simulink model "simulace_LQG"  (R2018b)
settings: Solver=ode4  StartTime=0.0  StopTime=10.5  FixedStep=1e-3  RelTol=1e-3
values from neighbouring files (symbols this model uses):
  b_0 = (bn_0 + bp_0) / 2    [mainSkript_simulaceLQG.m]    (also in mainSkript_rovniceSystemu.m = (params.bp_0 + params.bn_0) / 2; mainSkript_overeniRovnic.m = 0; mainSkript_LQGexperiment.m; mainSkript_LQGexperiment_integral.m)
  b_1 = params.b_1    [mainSkript_simulaceLQG.m]    (also in mainSkript_rovniceSystemu.m; mainSkript_overeniRovnic.m; mainSkript_kyvadlaNajednouOdhad.m; mainSkript_LQGexperiment.m)
  b_2 = params.b_2    [mainSkript_simulaceLQG.m]    (also in mainSkript_rovniceSystemu.m; mainSkript_overeniRovnic.m; mainSkript_kyvadlaNajednouOdhad.m; mainSkript_LQGexperiment.m)
  g = 9.81    [mainSkript_simulaceLQG.m]    (also in mainSkript_rovniceSystemu.m; mainSkript_overeniRovnic.m; mainSkript_estimaceVozik.m; mainSkript_odhadKyvadlaZvlast.m)
  I_1 = params.I_1    [mainSkript_simulaceLQG.m]    (also in mainSkript_rovniceSystemu.m; mainSkript_overeniRovnic.m; mainSkript_kyvadlaNajednouOdhad.m; mainSkript_LQGexperiment.m)
  I_2 = params.I_2    [mainSkript_simulaceLQG.m]    (also in mainSkript_rovniceSystemu.m; mainSkript_overeniRovnic.m; mainSkript_kyvadlaNajednouOdhad.m; mainSkript_LQGexperiment.m)
  K = lqr(sysd, Qk, Rk)    [mainSkript_simulaceLQG.m]    (also in makeFBL.m = [0; -d_2*g*sin(th_1); -d_3*g*sin(th_2)]; mainSkript_LQGexperiment.m = lqr(sysd, Q, R); mainSkript_LQGexperiment_integral.m = lqr(sysd, Q, R); mainSkript_pocitaniTVLQR_simplified.m = zeros(N + 1, n_sts))
  l_1 = params.l_1    [mainSkript_simulaceLQG.m]    (also in mainSkript_rovniceSystemu.m; mainSkript_overeniRovnic.m; odhadovane_parametry.m = 0.134; mainSkript_kyvadlaNajednouOdhad.m)
  L_1 = params.L_1    [mainSkript_simulaceLQG.m]    (also in mainSkript_rovniceSystemu.m; mainSkript_overeniRovnic.m; odhadovane_parametry.m = 0.228; mainSkript_kyvadlaNajednouOdhad.m)
  l_2 = params.l_2    [mainSkript_simulaceLQG.m]    (also in mainSkript_rovniceSystemu.m; mainSkript_overeniRovnic.m; odhadovane_parametry.m = 0.112; mainSkript_kyvadlaNajednouOdhad.m)
  m_0 = params.m_0    [mainSkript_simulaceLQG.m]    (also in mainSkript_rovniceSystemu.m; mainSkript_overeniRovnic.m; mainSkript_LQGexperiment.m; mainSkript_LQGexperiment_integral.m)
  m_1 = params.m_1    [mainSkript_simulaceLQG.m]    (also in mainSkript_rovniceSystemu.m; mainSkript_overeniRovnic.m; mainSkript_kyvadlaNajednouOdhad.m; mainSkript_LQGexperiment.m)
  m_2 = params.m_2    [mainSkript_simulaceLQG.m]    (also in mainSkript_rovniceSystemu.m; mainSkript_overeniRovnic.m; mainSkript_kyvadlaNajednouOdhad.m; mainSkript_LQGexperiment.m)
  N = N * Cref'    [mainSkript_simulaceLQG.m]    (also in mainSkript_tvorbaTrajektorii.m = 100; mainSkript_pocitaniTVLQR_simplified.m = floor( length(time) / krok ))
  q_0 = [0 th1_0 th2_0 0 dth1_0 dth2_0]    [mainSkript_simulaceLQG.m]    (also in mainSkript_kyvadlaNajednouOdhad.m = cell(1, k); mainSkript_LQGexperiment.m = zeros(6,1); mainSkript_LQGexperiment_integral.m = zeros(6,1); mainSkript_modifikaceParametru.m = [0 pi pi 0 0 0])
  Ts = 1e-3    (= 0.001)    [mainSkript_simulaceLQG.m]    (also in mainSkript_rovniceSystemu.m; mainSkript_LQGexperiment.m; mainSkript_LQGexperiment_integral.m; mainSkript_modifikaceParametru.m)
undefined symbols (not defined in the file or in its folder): DiscIntNeverNeededParam
libraries: sharedTrackingLibrary x1, simulink x1

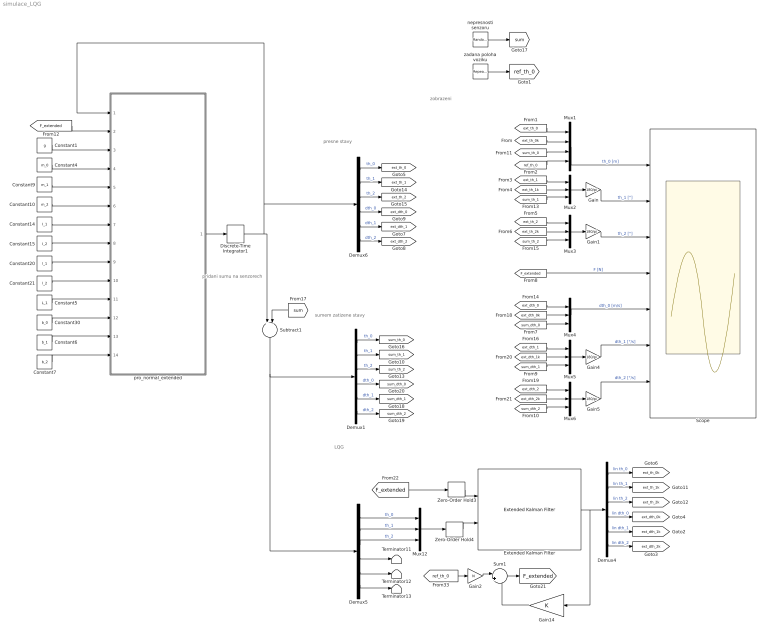
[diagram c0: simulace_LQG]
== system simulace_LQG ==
  note: sumem zatizene stavy
  note: presne stavy
  note: zobrazeni
  note: pridani sumu na senzorech
  note: LQG
  Constant1 : Constant  Value=g
  Constant10 : Constant  Value=m_2
  Constant14 : Constant  Value=I_1
  Constant15 : Constant  Value=I_2
  Constant20 : Constant  Value=l_1
  Constant21 : Constant  Value=l_2
  Constant30 : Constant  Value=b_0
  Constant4 : Constant  Value=m_0
  Constant5 : Constant  Value=L_1
  Constant6 : Constant  Value=b_1
  Constant7 : Constant  Value=b_2
  Constant9 : Constant  Value=m_1
  Demux{1,4..6} (4 alike) : Demux  Outputs=6
  Discrete-Time Integrator1 : DiscreteIntegrator  InitialCondition=q_0  SampleTime=Ts  ICPrevOutput=DiscIntNeverNeededParam  ICPrevScaledInput=DiscIntNeverNeededParam
  Extended Kalman Filter : sharedTrackingLibrary/Extended Kalman Filter  StateTransitionFcn=nonLinKalmFcn  HasStateTransitionJacobianFcn=on  StateTransitionJacobianFcn=countJacobDIP  HasAdditiveProcessNoise=Additive  ProcessNoise=Q_kalm  HasTimeVaryingProcessNoise=off  HasStateTransitionFcnExtraArgument=1  InitialState=q_0  InitialStateCovariance=1e-3*eye(6)  MeasurementFcn1=mereniStavuKalm  HasMeasurementJacobianFcn1=off  HasMeasurementEnablePort1=off  HasAdditiveMeasurementNoise1=Additive  MeasurementNoise1=R_kalm  HasTimeVaryingMeasurementNoise1=off  HasMeasurementFcnExtraArgument1=0  MeasurementFcn2=myMeasurementFcn  HasMeasurementJacobianFcn2=off  HasMeasurementEnablePort2=off  HasAdditiveMeasurementNoise2=Additive  MeasurementNoise2=1  HasTimeVaryingMeasurementNoise2=off  HasMeasurementFcnExtraArgument2=0  MeasurementFcn3=myMeasurementFcn  HasMeasurementJacobianFcn3=off  HasMeasurementEnablePort3=off  HasAdditiveMeasurementNoise3=Additive  MeasurementNoise3=1  HasTimeVaryingMeasurementNoise3=off  HasMeasurementFcnExtraArgument3=0  MeasurementFcn4=myMeasurementFcn  HasMeasurementJacobianFcn4=off  HasMeasurementEnablePort4=off  HasAdditiveMeasurementNoise4=Additive  MeasurementNoise4=1  HasTimeVaryingMeasurementNoise4=off  HasMeasurementFcnExtraArgument4=0  MeasurementFcn5=myMeasurementFcn  HasMeasurementJacobianFcn5=off  HasMeasurementEnablePort5=off  HasAdditiveMeasurementNoise5=Additive  MeasurementNoise5=1  HasTimeVaryingMeasurementNoise5=off  HasMeasurementFcnExtraArgument5=0  EnableMultirate=off  StateTransitionFcnSampleTime=1  MeasurementFcn1SampleTime=1  MeasurementFcn2SampleTime=1  MeasurementFcn3SampleTime=1  MeasurementFcn4SampleTime=1  MeasurementFcn5SampleTime=1  UseCurrentEstimator=on  OutputStateCovariance=off  DataType=double  SampleTime=1e-3  NumberOfMeasurements=1
  Gain{,1,4..5} (4 alike) : Gain  Gain=180/pi
  Gain14 : Gain  Gain=K  Multiplication=Matrix(K*u) (u vector)
  Gain2 : Gain  Gain=N
  Mux1 : Mux
  Mux{2..6,12} (6 alike) : Mux  Inputs=3
  Scope : Scope  NumInputPorts=7
  Subtract1 : Sum  Inputs=+-
  Sum1 : Sum  Inputs=|+-
  Terminator11 : Terminator
  Terminator12 : Terminator
  Terminator13 : Terminator
  Zero-Order Hold3 : ZeroOrderHold  SampleTime=1e-3
  Zero-Order Hold4 : ZeroOrderHold  SampleTime=1e-3
  nepresnosti senzoru : RandomNumber  Mean=zeros(6,1)  Variance=[1e-5 .* ones(6,1)]  SampleTime=1e-3
  pro_normal_extended : MATLAB Function  TreatAsAtomicUnit=on
  zadana poloha voziku : simulink/Sources/Repeating Sequence Stair  OutValues=[0 0.1 -0.1]  tsamp=5  OutMin=[]  OutMax=[]  OutDataTypeStr=double  OutputDataTypeScalingMode=double  OutDataType=fixdt(0,8)  ConRadixGroup=Best Precision: Vector-wise  OutScaling=2^-12
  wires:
  [F_extended] -> Zero-Order Hold3/1
  Demux4/1 -> [ext_th_0k]  "lin th_0"
  Demux4/4 -> [ext_dth_0k]  "lin dth_0"
  Demux4/5 -> [ext_dth_1k]  "lin dth_1"
  Demux4/3 -> [ext_th_2k]  "lin th_2"
  Demux4/2 -> [ext_th_1k]  "lin th_1"
  Demux4/6 -> [ext_dth_2k]  "lin dth_2"
  Extended Kalman Filter/1 -> Gain14/1, Demux4/1
  Constant30/1 -> pro_normal_extended/12(b_0)
  Constant7/1 -> pro_normal_extended/14(b_2)
  Constant5/1 -> pro_normal_extended/11(L_1)
  Demux6/2 -> [ext_th_1]  "th_1"
  Constant1/1 -> pro_normal_extended/3(g)
  Constant21/1 -> pro_normal_extended/10(l_2)
  Demux6/3 -> [ext_th_2]  "th_2"
  Constant6/1 -> pro_normal_extended/13(b_1)
  Demux6/1 -> [ext_th_0]  "th_0"
  pro_normal_extended/1(dx) -> Discrete-Time Integrator1/1
  Constant14/1 -> pro_normal_extended/7(I_1)
  Constant15/1 -> pro_normal_extended/8(I_2)
  Constant4/1 -> pro_normal_extended/4(m_0)
  Constant9/1 -> pro_normal_extended/5(m_1)
  Constant20/1 -> pro_normal_extended/9(l_1)
  Discrete-Time Integrator1/1 -> Demux6/1, pro_normal_extended/1(y), Subtract1/1
  Constant10/1 -> pro_normal_extended/6(m_2)
  [F_extended] -> pro_normal_extended/2(u)
  nepresnosti senzoru/1 -> [sum]
  [sum] -> Subtract1/2
  zadana poloha voziku/1 -> [ref_th_0]
  [ext_th_1] -> Mux2/1
  [ext_th_1k] -> Mux2/2
  [ext_th_2k] -> Mux3/2
  [ext_th_2] -> Mux3/1
  Mux1/1 -> Scope/1  "th_0 [m]"
  Mux2/1 -> Gain/1
  Mux3/1 -> Gain1/1
  [F_extended] -> Scope/4  "F [N]"
  Gain/1 -> Scope/2  "th_1 [°]"
  Gain1/1 -> Scope/3  "th_2 [°]"
  [ext_th_0] -> Mux1/1
  [ext_th_0k] -> Mux1/2
  [ref_th_0] -> Gain2/1
  Gain2/1 -> Sum1/1
  Gain14/1 -> Sum1/2
  Zero-Order Hold3/1 -> Extended Kalman Filter/1
  Zero-Order Hold4/1 -> Extended Kalman Filter/2
  Mux6/1 -> Gain5/1
  Gain4/1 -> Scope/6  "dth_1 [°/s]"
  Gain5/1 -> Scope/7  "dth_2 [°/s]"
  Demux6/4 -> [ext_dth_0]  "dth_0"
  Demux6/5 -> [ext_dth_1]  "dth_1"
  Demux6/6 -> [ext_dth_2]  "dth_2"
  Mux4/1 -> Scope/5  "dth_0 [m/s]"
  Demux1/6 -> [sum_dth_2]  "dth_2"
  Demux1/5 -> [sum_dth_1]  "dth_1"
  Demux1/4 -> [sum_dth_0]  "dth_0"
  Demux1/1 -> [sum_th_0]  "th_0"
  Demux1/3 -> [sum_th_2]  "th_2"
  Demux1/2 -> [sum_th_1]  "th_1"
  [ref_th_0] -> Mux1/4
  [sum_th_0] -> Mux1/3
  [sum_th_1] -> Mux2/3
  [sum_th_2] -> Mux3/3
  [ext_dth_0] -> Mux4/1
  [sum_dth_0] -> Mux4/3
  [ext_dth_0k] -> Mux4/2
  [ext_dth_1] -> Mux5/1
  [sum_dth_1] -> Mux5/3
  [ext_dth_1k] -> Mux5/2
  Mux5/1 -> Gain4/1
  [ext_dth_2] -> Mux6/1
  [sum_dth_2] -> Mux6/3
  [ext_dth_2k] -> Mux6/2
  Sum1/1 -> [F_extended]
  Demux5/2 -> Mux12/2  "th_1"
  Demux5/3 -> Mux12/3  "th_2"
  Demux5/6 -> Terminator13/1
  Demux5/1 -> Mux12/1  "th_0"
  Demux5/4 -> Terminator11/1
  Demux5/5 -> Terminator12/1
  Mux12/1 -> Zero-Order Hold4/1
  Subtract1/1 -> Demux5/1, Demux1/1

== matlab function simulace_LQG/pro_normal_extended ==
function dx = PohybovaRceDIP_basic(y, u, g, m_0, m_1, m_2, I_1, I_2, l_1, l_2, L_1, b_0, b_1, b_2)
%PohybovaRceDIP_basic: Pohybova rovnice dvojiteho kyvadla

dx = zeros(6, 1); % definovani sloupcoveho vektoru derivaci stavu 

dx(1) = conj(y(4)); 
dx(2) = conj(y(5)); 
dx(3) = conj(y(6)); 
dx(4) = conj(y(6))*((b_2*(L_1^2*l_2*m_2^2*cos(y(3)) + I_1*l_2*m_2*cos(y(3)) - L_1^2*l_2*m_2^2*cos(y(2) - y(3))*cos(y(2)) + l_1^2*l_2*m_1*m_2*cos(y(3)) - L_1*l_1*l_2*m_1*m_2*cos(y(2) - y(3))*cos(y(2))))/(I_2*L_1^2*m_2^2 + I_2*l_1^2*m_1^2 + I_1*l_2^2*m_2^2 + I_1*I_2*m_0 + I_1*I_2*m_1 + I_1*I_2*m_2 + L_1^2*l_2^2*m_2^3 + L_1^2*l_2^2*m_0*m_2^2 + L_1^2*l_2^2*m_1*m_2^2 - L_1^2*l_2^2*m_2^3*cos(y(2) - y(3))^2 + I_2*L_1^2*m_0*m_2 + I_2*L_1^2*m_1*m_2 + l_1^2*l_2^2*m_1*m_2^2 + l_1^2*l_2^2*m_1^2*m_2 + I_2*l_1^2*m_0*m_1 + I_1*l_2^2*m_0*m_2 + I_1*l_2^2*m_1*m_2 + I_2*l_1^2*m_1*m_2 - I_2*L_1^2*m_2^2*cos(y(2))^2 - I_2*l_1^2*m_1^2*cos(y(2))^2 - I_1*l_2^2*m_2^2*cos(y(3))^2 - L_1^2*l_2^2*m_2^3*cos(y(2))^2 - L_1^2*l_2^2*m_2^3*cos(y(3))^2 + l_1^2*l_2^2*m_0*m_1*m_2 - l_1^2*l_2^2*m_1^2*m_2*cos(y(2))^2 - l_1^2*l_2^2*m_1*m_2^2*cos(y(3))^2 - L_1^2*l_2^2*m_0*m_2^2*cos(y(2) - y(3))^2 - L_1^2*l_2^2*m_1*m_2^2*cos(y(2) - y(3))^2 - 2*L_1*l_1*l_2^2*m_1*m_2^2*cos(y(2))^2 + 2*L_1^2*l_2^2*m_2^3*cos(y(2) - y(3))*cos(y(2))*cos(y(3)) - 2*I_2*L_1*l_1*m_1*m_2*cos(y(2))^2 + 2*L_1*l_1*l_2^2*m_1*m_2^2*cos(y(2) - y(3))*cos(y(2))*cos(y(3))) - ((b_2 - L_1*l_2*m_2*sin(y(2) - y(3))*y(6))*(L_1*l_2^2*m_2^2*cos(y(2)) + I_2*L_1*m_2*cos(y(2)) + I_2*l_1*m_1*cos(y(2)) - L_1*l_2^2*m_2^2*cos(y(2) - y(3))*cos(y(3)) + l_1*l_2^2*m_1*m_2*cos(y(2))))/(I_2*L_1^2*m_2^2 + I_2*l_1^2*m_1^2 + I_1*l_2^2*m_2^2 + I_1*I_2*m_0 + I_1*I_2*m_1 + I_1*I_2*m_2 + L_1^2*l_2^2*m_2^3 + L_1^2*l_2^2*m_0*m_2^2 + L_1^2*l_2^2*m_1*m_2^2 - L_1^2*l_2^2*m_2^3*cos(y(2) - y(3))^2 + I_2*L_1^2*m_0*m_2 + I_2*L_1^2*m_1*m_2 + l_1^2*l_2^2*m_1*m_2^2 + l_1^2*l_2^2*m_1^2*m_2 + I_2*l_1^2*m_0*m_1 + I_1*l_2^2*m_0*m_2 + I_1*l_2^2*m_1*m_2 + I_2*l_1^2*m_1*m_2 - I_2*L_1^2*m_2^2*cos(y(2))^2 - I_2*l_1^2*m_1^2*cos(y(2))^2 - I_1*l_2^2*m_2^2*cos(y(3))^2 - L_1^2*l_2^2*m_2^3*cos(y(2))^2 - L_1^2*l_2^2*m_2^3*cos(y(3))^2 + l_1^2*l_2^2*m_0*m_1*m_2 - l_1^2*l_2^2*m_1^2*m_2*cos(y(2))^2 - l_1^2*l_2^2*m_1*m_2^2*cos(y(3))^2 - L_1^2*l_2^2*m_0*m_2^2*cos(y(2) - y(3))^2 - L_1^2*l_2^2*m_1*m_2^2*cos(y(2) - y(3))^2 - 2*L_1*l_1*l_2^2*m_1*m_2^2*cos(y(2))^2 + 2*L_1^2*l_2^2*m_2^3*cos(y(2) - y(3))*cos(y(2))*cos(y(3)) - 2*I_2*L_1*l_1*m_1*m_2*cos(y(2))^2 + 2*L_1*l_1*l_2^2*m_1*m_2^2*cos(y(2) - y(3))*cos(y(2))*cos(y(3))) + (l_2*m_2*y(6)*sin(y(3))*(I_1*I_2 + L_1^2*l_2^2*m_2^2 + I_2*L_1^2*m_2 + I_2*l_1^2*m_1 + I_1*l_2^2*m_2 - L_1^2*l_2^2*m_2^2*cos(y(2) - y(3))^2 + l_1^2*l_2^2*m_1*m_2))/(I_2*L_1^2*m_2^2 + I_2*l_1^2*m_1^2 + I_1*l_2^2*m_2^2 + I_1*I_2*m_0 + I_1*I_2*m_1 + I_1*I_2*m_2 + L_1^2*l_2^2*m_2^3 + L_1^2*l_2^2*m_0*m_2^2 + L_1^2*l_2^2*m_1*m_2^2 - L_1^2*l_2^2*m_2^3*cos(y(2) - y(3))^2 + I_2*L_1^2*m_0*m_2 + I_2*L_1^2*m_1*m_2 + l_1^2*l_2^2*m_1*m_2^2 + l_1^2*l_2^2*m_1^2*m_2 + I_2*l_1^2*m_0*m_1 + I_1*l_2^2*m_0*m_2 + I_1*l_2^2*m_1*m_2 + I_2*l_1^2*m_1*m_2 - I_2*L_1^2*m_2^2*cos(y(2))^2 - I_2*l_1^2*m_1^2*cos(y(2))^2 - I_1*l_2^2*m_2^2*cos(y(3))^2 - L_1^2*l_2^2*m_2^3*cos(y(2))^2 - L_1^2*l_2^2*m_2^3*cos(y(3))^2 + l_1^2*l_2^2*m_0*m_1*m_2 - l_1^2*l_2^2*m_1^2*m_2*cos(y(2))^2 - l_1^2*l_2^2*m_1*m_2^2*cos(y(3))^2 - L_1^2*l_2^2*m_0*m_2^2*cos(y(2) - y(3))^2 - L_1^2*l_2^2*m_1*m_2^2*cos(y(2) - y(3))^2 - 2*L_1*l_1*l_2^2*m_1*m_2^2*cos(y(2))^2 + 2*L_1^2*l_2^2*m_2^3*cos(y(2) - y(3))*cos(y(2))*cos(y(3)) - 2*I_2*L_1*l_1*m_1*m_2*cos(y(2))^2 + 2*L_1*l_1*l_2^2*m_1*m_2^2*cos(y(2) - y(3))*cos(y(2))*cos(y(3)))) + conj(y(5))*(((b_1 + b_2)*(L_1*l_2^2*m_2^2*cos(y(2)) + I_2*L_1*m_2*cos(y(2)) + I_2*l_1*m_1*cos(y(2)) - L_1*l_2^2*m_2^2*cos(y(2) - y(3))*cos(y(3)) + l_1*l_2^2*m_1*m_2*cos(y(2))))/(I_2*L_1^2*m_2^2 + I_2*l_1^2*m_1^2 + I_1*l_2^2*m_2^2 + I_1*I_2*m_0 + I_1*I_2*m_1 + I_1*I_2*m_2 + L_1^2*l_2^2*m_2^3 + L_1^2*l_2^2*m_0*m_2^2 + L_1^2*l_2^2*m_1*m_2^2 - L_1^2*l_2^2*m_2^3*cos(y(2) - y(3))^2 + I_2*L_1^2*m_0*m_2 + I_2*L_1^2*m_1*m_2 + l_1^2*l_2^2*m_1*m_2^2 + l_1^2*l_2^2*m_1^2*m_2 + I_2*l_1^2*m_0*m_1 + I_1*l_2^2*m_0*m_2 + I_1*l_2^2*m_1*m_2 + I_2*l_1^2*m_1*m_2 - I_2*L_1^2*m_2^2*cos(y(2))^2 - I_2*l_1^2*m_1^2*cos(y(2))^2 - I_1*l_2^2*m_2^2*cos(y(3))^2 - L_1^2*l_2^2*m_2^3*cos(y(2))^2 - L_1^2*l_2^2*m_2^3*cos(y(3))^2 + l_1^2*l_2^2*m_0*m_1*m_2 - l_1^2*l_2^2*m_1^2*m_2*cos(y(2))^2 - l_1^2*l_2^2*m_1*m_2^2*cos(y(3))^2 - L_1^2*l_2^2*m_0*m_2^2*cos(y(2) - y(3))^2 - L_1^2*l_2^2*m_1*m_2^2*cos(y(2) - y(3))^2 - 2*L_1*l_1*l_2^2*m_1*m_2^2*cos(y(2))^2 + 2*L_1^2*l_2^2*m_2^3*cos(y(2) - y(3))*cos(y(2))*cos(y(3)) - 2*I_2*L_1*l_1*m_1*m_2*cos(y(2))^2 + 2*L_1*l_1*l_2^2*m_1*m_2^2*cos(y(2) - y(3))*cos(y(2))*cos(y(3))) - ((b_2 + L_1*l_2*m_2*sin(y(2) - y(3))*y(5))*(L_1^2*l_2*m_2^2*cos(y(3)) + I_1*l_2*m_2*cos(y(3)) - L_1^2*l_2*m_2^2*cos(y(2) - y(3))*cos(y(2)) + l_1^2*l_2*m_1*m_2*cos(y(3)) - L_1*l_1*l_2*m_1*m_2*cos(y(2) - y(3))*cos(y(2))))/(I_2*L_1^2*m_2^2 + I_2*l_1^2*m_1^2 + I_1*l_2^2*m_2^2 + I_1*I_2*m_0 + I_1*I_2*m_1 + I_1*I_2*m_2 + L_1^2*l_2^2*m_2^3 + L_1^2*l_2^2*m_0*m_2^2 + L_1^2*l_2^2*m_1*m_2^2 - L_1^2*l_2^2*m_2^3*cos(y(2) - y(3))^2 + I_2*L_1^2*m_0*m_2 + I_2*L_1^2*m_1*m_2 + l_1^2*l_2^2*m_1*m_2^2 + l_1^2*l_2^2*m_1^2*m_2 + I_2*l_1^2*m_0*m_1 + I_1*l_2^2*m_0*m_2 + I_1*l_2^2*m_1*m_2 + I_2*l_1^2*m_1*m_2 - I_2*L_1^2*m_2^2*cos(y(2))^2 - I_2*l_1^2*m_1^2*cos(y(2))^2 - I_1*l_2^2*m_2^2*cos(y(3))^2 - L_1^2*l_2^2*m_2^3*cos(y(2))^2 - L_1^2*l_2^2*m_2^3*cos(y(3))^2 + l_1^2*l_2^2*m_0*m_1*m_2 - l_1^2*l_2^2*m_1^2*m_2*cos(y(2))^2 - l_1^2*l_2^2*m_1*m_2^2*cos(y(3))^2 - L_1^2*l_2^2*m_0*m_2^2*cos(y(2) - y(3))^2 - L_1^2*l_2^2*m_1*m_2^2*cos(y(2) - y(3))^2 - 2*L_1*l_1*l_2^2*m_1*m_2^2*cos(y(2))^2 + 2*L_1^2*l_2^2*m_2^3*cos(y(2) - y(3))*cos(y(2))*cos(y(3)) - 2*I_2*L_1*l_1*m_1*m_2*cos(y(2))^2 + 2*L_1*l_1*l_2^2*m_1*m_2^2*cos(y(2) - y(3))*cos(y(2))*cos(y(3))) + (y(5)*sin(y(2))*(L_1*m_2 + l_1*m_1)*(I_1*I_2 + L_1^2*l_2^2*m_2^2 + I_2*L_1^2*m_2 + I_2*l_1^2*m_1 + I_1*l_2^2*m_2 - L_1^2*l_2^2*m_2^2*cos(y(2) - y(3))^2 + l_1^2*l_2^2*m_1*m_2))/(I_2*L_1^2*m_2^2 + I_2*l_1^2*m_1^2 + I_1*l_2^2*m_2^2 + I_1*I_2*m_0 + I_1*I_2*m_1 + I_1*I_2*m_2 + L_1^2*l_2^2*m_2^3 + L_1^2*l_2^2*m_0*m_2^2 + L_1^2*l_2^2*m_1*m_2^2 - L_1^2*l_2^2*m_2^3*cos(y(2) - y(3))^2 + I_2*L_1^2*m_0*m_2 + I_2*L_1^2*m_1*m_2 + l_1^2*l_2^2*m_1*m_2^2 + l_1^2*l_2^2*m_1^2*m_2 + I_2*l_1^2*m_0*m_1 + I_1*l_2^2*m_0*m_2 + I_1*l_2^2*m_1*m_2 + I_2*l_1^2*m_1*m_2 - I_2*L_1^2*m_2^2*cos(y(2))^2 - I_2*l_1^2*m_1^2*cos(y(2))^2 - I_1*l_2^2*m_2^2*cos(y(3))^2 - L_1^2*l_2^2*m_2^3*cos(y(2))^2 - L_1^2*l_2^2*m_2^3*cos(y(3))^2 + l_1^2*l_2^2*m_0*m_1*m_2 - l_1^2*l_2^2*m_1^2*m_2*cos(y(2))^2 - l_1^2*l_2^2*m_1*m_2^2*cos(y(3))^2 - L_1^2*l_2^2*m_0*m_2^2*cos(y(2) - y(3))^2 - L_1^2*l_2^2*m_1*m_2^2*cos(y(2) - y(3))^2 - 2*L_1*l_1*l_2^2*m_1*m_2^2*cos(y(2))^2 + 2*L_1^2*l_2^2*m_2^3*cos(y(2) - y(3))*cos(y(2))*cos(y(3)) - 2*I_2*L_1*l_1*m_1*m_2*cos(y(2))^2 + 2*L_1*l_1*l_2^2*m_1*m_2^2*cos(y(2) - y(3))*cos(y(2))*cos(y(3)))) + (u*(I_1*I_2 + L_1^2*l_2^2*m_2^2 + I_2*L_1^2*m_2 + I_2*l_1^2*m_1 + I_1*l_2^2*m_2 - L_1^2*l_2^2*m_2^2*cos(y(2) - y(3))^2 + l_1^2*l_2^2*m_1*m_2))/(I_2*L_1^2*m_2^2 + I_2*l_1^2*m_1^2 + I_1*l_2^2*m_2^2 + I_1*I_2*m_0 + I_1*I_2*m_1 + I_1*I_2*m_2 + L_1^2*l_2^2*m_2^3 + L_1^2*l_2^2*m_0*m_2^2 + L_1^2*l_2^2*m_1*m_2^2 - L_1^2*l_2^2*m_2^3*cos(y(2) - y(3))^2 + I_2*L_1^2*m_0*m_2 + I_2*L_1^2*m_1*m_2 + l_1^2*l_2^2*m_1*m_2^2 + l_1^2*l_2^2*m_1^2*m_2 + I_2*l_1^2*m_0*m_1 + I_1*l_2^2*m_0*m_2 + I_1*l_2^2*m_1*m_2 + I_2*l_1^2*m_1*m_2 - I_2*L_1^2*m_2^2*cos(y(2))^2 - I_2*l_1^2*m_1^2*cos(y(2))^2 - I_1*l_2^2*m_2^2*cos(y(3))^2 - L_1^2*l_2^2*m_2^3*cos(y(2))^2 - L_1^2*l_2^2*m_2^3*cos(y(3))^2 + l_1^2*l_2^2*m_0*m_1*m_2 - l_1^2*l_2^2*m_1^2*m_2*cos(y(2))^2 - l_1^2*l_2^2*m_1*m_2^2*cos(y(3))^2 - L_1^2*l_2^2*m_0*m_2^2*cos(y(2) - y(3))^2 - L_1^2*l_2^2*m_1*m_2^2*cos(y(2) - y(3))^2 - 2*L_1*l_1*l_2^2*m_1*m_2^2*cos(y(2))^2 + 2*L_1^2*l_2^2*m_2^3*cos(y(2) - y(3))*cos(y(2))*cos(y(3)) - 2*I_2*L_1*l_1*m_1*m_2*cos(y(2))^2 + 2*L_1*l_1*l_2^2*m_1*m_2^2*cos(y(2) - y(3))*cos(y(2))*cos(y(3))) - (b_0*conj(y(4))*(I_1*I_2 + L_1^2*l_2^2*m_2^2 + I_2*L_1^2*m_2 + I_2*l_1^2*m_1 + I_1*l_2^2*m_2 - L_1^2*l_2^2*m_2^2*cos(y(2) - y(3))^2 + l_1^2*l_2^2*m_1*m_2))/(I_2*L_1^2*m_2^2 + I_2*l_1^2*m_1^2 + I_1*l_2^2*m_2^2 + I_1*I_2*m_0 + I_1*I_2*m_1 + I_1*I_2*m_2 + L_1^2*l_2^2*m_2^3 + L_1^2*l_2^2*m_0*m_2^2 + L_1^2*l_2^2*m_1*m_2^2 - L_1^2*l_2^2*m_2^3*cos(y(2) - y(3))^2 + I_2*L_1^2*m_0*m_2 + I_2*L_1^2*m_1*m_2 + l_1^2*l_2^2*m_1*m_2^2 + l_1^2*l_2^2*m_1^2*m_2 + I_2*l_1^2*m_0*m_1 + I_1*l_2^2*m_0*m_2 + I_1*l_2^2*m_1*m_2 + I_2*l_1^2*m_1*m_2 - I_2*L_1^2*m_2^2*cos(y(2))^2 - I_2*l_1^2*m_1^2*cos(y(2))^2 - I_1*l_2^2*m_2^2*cos(y(3))^2 - L_1^2*l_2^2*m_2^3*cos(y(2))^2 - L_1^2*l_2^2*m_2^3*cos(y(3))^2 + l_1^2*l_2^2*m_0*m_1*m_2 - l_1^2*l_2^2*m_1^2*m_2*cos(y(2))^2 - l_1^2*l_2^2*m_1*m_2^2*cos(y(3))^2 - L_1^2*l_2^2*m_0*m_2^2*cos(y(2) - y(3))^2 - L_1^2*l_2^2*m_1*m_2^2*cos(y(2) - y(3))^2 - 2*L_1*l_1*l_2^2*m_1*m_2^2*cos(y(2))^2 + 2*L_1^2*l_2^2*m_2^3*cos(y(2) - y(3))*cos(y(2))*cos(y(3)) - 2*I_2*L_1*l_1*m_1*m_2*cos(y(2))^2 + 2*L_1*l_1*l_2^2*m_1*m_2^2*cos(y(2) - y(3))*cos(y(2))*cos(y(3))) - (g*sin(y(2))*(L_1*m_2 + l_1*m_1)*(L_1*l_2^2*m_2^2*cos(y(2)) + I_2*L_1*m_2*cos(y(2)) + I_2*l_1*m_1*cos(y(2)) - L_1*l_2^2*m_2^2*cos(y(2) - y(3))*cos(y(3)) + l_1*l_2^2*m_1*m_2*cos(y(2))))/(I_2*L_1^2*m_2^2 + I_2*l_1^2*m_1^2 + I_1*l_2^2*m_2^2 + I_1*I_2*m_0 + I_1*I_2*m_1 + I_1*I_2*m_2 + L_1^2*l_2^2*m_2^3 + L_1^2*l_2^2*m_0*m_2^2 + L_1^2*l_2^2*m_1*m_2^2 - L_1^2*l_2^2*m_2^3*cos(y(2) - y(3))^2 + I_2*L_1^2*m_0*m_2 + I_2*L_1^2*m_1*m_2 + l_1^2*l_2^2*m_1*m_2^2 + l_1^2*l_2^2*m_1^2*m_2 + I_2*l_1^2*m_0*m_1 + I_1*l_2^2*m_0*m_2 + I_1*l_2^2*m_1*m_2 + I_2*l_1^2*m_1*m_2 - I_2*L_1^2*m_2^2*cos(y(2))^2 - I_2*l_1^2*m_1^2*cos(y(2))^2 - I_1*l_2^2*m_2^2*cos(y(3))^2 - L_1^2*l_2^2*m_2^3*cos(y(2))^2 - L_1^2*l_2^2*m_2^3*cos(y(3))^2 + l_1^2*l_2^2*m_0*m_1*m_2 - l_1^2*l_2^2*m_1^2*m_2*cos(y(2))^2 - l_1^2*l_2^2*m_1*m_2^2*cos(y(3))^2 - L_1^2*l_2^2*m_0*m_2^2*cos(y(2) - y(3))^2 - L_1^2*l_2^2*m_1*m_2^2*cos(y(2) - y(3))^2 - 2*L_1*l_1*l_2^2*m_1*m_2^2*cos(y(2))^2 + 2*L_1^2*l_2^2*m_2^3*cos(y(2) - y(3))*cos(y(2))*cos(y(3)) - 2*I_2*L_1*l_1*m_1*m_2*cos(y(2))^2 + 2*L_1*l_1*l_2^2*m_1*m_2^2*cos(y(2) - y(3))*cos(y(2))*cos(y(3))) - (g*l_2*m_2*sin(y(3))*(L_1^2*l_2*m_2^2*cos(y(3)) + I_1*l_2*m_2*cos(y(3)) - L_1^2*l_2*m_2^2*cos(y(2) - y(3))*cos(y(2)) + l_1^2*l_2*m_1*m_2*cos(y(3)) - L_1*l_1*l_2*m_1*m_2*cos(y(2) - y(3))*cos(y(2))))/(I_2*L_1^2*m_2^2 + I_2*l_1^2*m_1^2 + I_1*l_2^2*m_2^2 + I_1*I_2*m_0 + I_1*I_2*m_1 + I_1*I_2*m_2 + L_1^2*l_2^2*m_2^3 + L_1^2*l_2^2*m_0*m_2^2 + L_1^2*l_2^2*m_1*m_2^2 - L_1^2*l_2^2*m_2^3*cos(y(2) - y(3))^2 + I_2*L_1^2*m_0*m_2 + I_2*L_1^2*m_1*m_2 + l_1^2*l_2^2*m_1*m_2^2 + l_1^2*l_2^2*m_1^2*m_2 + I_2*l_1^2*m_0*m_1 + I_1*l_2^2*m_0*m_2 + I_1*l_2^2*m_1*m_2 + I_2*l_1^2*m_1*m_2 - I_2*L_1^2*m_2^2*cos(y(2))^2 - I_2*l_1^2*m_1^2*cos(y(2))^2 - I_1*l_2^2*m_2^2*cos(y(3))^2 - L_1^2*l_2^2*m_2^3*cos(y(2))^2 - L_1^2*l_2^2*m_2^3*cos(y(3))^2 + l_1^2*l_2^2*m_0*m_1*m_2 - l_1^2*l_2^2*m_1^2*m_2*cos(y(2))^2 - l_1^2*l_2^2*m_1*m_2^2*cos(y(3))^2 - L_1^2*l_2^2*m_0*m_2^2*cos(y(2) - y(3))^2 - L_1^2*l_2^2*m_1*m_2^2*cos(y(2) - y(3))^2 - 2*L_1*l_1*l_2^2*m_1*m_2^2*cos(y(2))^2 + 2*L_1^2*l_2^2*m_2^3*cos(y(2) - y(3))*cos(y(2))*cos(y(3)) - 2*I_2*L_1*l_1*m_1*m_2*cos(y(2))^2 + 2*L_1*l_1*l_2^2*m_1*m_2^2*cos(y(2) - y(3))*cos(y(2))*cos(y(3))); 
dx(5) = conj(y(6))*((b_2*(L_1*l_2*m_2^2*cos(y(2) - y(3)) + L_1*l_2*m_0*m_2*cos(y(2) - y(3)) + L_1*l_2*m_1*m_2*cos(y(2) - y(3)) - L_1*l_2*m_2^2*cos(y(2))*cos(y(3)) - l_1*l_2*m_1*m_2*cos(y(2))*cos(y(3))))/(I_2*L_1^2*m_2^2 + I_2*l_1^2*m_1^2 + I_1*l_2^2*m_2^2 + I_1*I_2*m_0 + I_1*I_2*m_1 + I_1*I_2*m_2 + L_1^2*l_2^2*m_2^3 + L_1^2*l_2^2*m_0*m_2^2 + L_1^2*l_2^2*m_1*m_2^2 - L_1^2*l_2^2*m_2^3*cos(y(2) - y(3))^2 + I_2*L_1^2*m_0*m_2 + I_2*L_1^2*m_1*m_2 + l_1^2*l_2^2*m_1*m_2^2 + l_1^2*l_2^2*m_1^2*m_2 + I_2*l_1^2*m_0*m_1 + I_1*l_2^2*m_0*m_2 + I_1*l_2^2*m_1*m_2 + I_2*l_1^2*m_1*m_2 - I_2*L_1^2*m_2^2*cos(y(2))^2 - I_2*l_1^2*m_1^2*cos(y(2))^2 - I_1*l_2^2*m_2^2*cos(y(3))^2 - L_1^2*l_2^2*m_2^3*cos(y(2))^2 - L_1^2*l_2^2*m_2^3*cos(y(3))^2 + l_1^2*l_2^2*m_0*m_1*m_2 - l_1^2*l_2^2*m_1^2*m_2*cos(y(2))^2 - l_1^2*l_2^2*m_1*m_2^2*cos(y(3))^2 - L_1^2*l_2^2*m_0*m_2^2*cos(y(2) - y(3))^2 - L_1^2*l_2^2*m_1*m_2^2*cos(y(2) - y(3))^2 - 2*L_1*l_1*l_2^2*m_1*m_2^2*cos(y(2))^2 + 2*L_1^2*l_2^2*m_2^3*cos(y(2) - y(3))*cos(y(2))*cos(y(3)) - 2*I_2*L_1*l_1*m_1*m_2*cos(y(2))^2 + 2*L_1*l_1*l_2^2*m_1*m_2^2*cos(y(2) - y(3))*cos(y(2))*cos(y(3))) + ((b_2 - L_1*l_2*m_2*sin(y(2) - y(3))*y(6))*(I_2*m_0 + I_2*m_1 + I_2*m_2 + l_2^2*m_2^2 + l_2^2*m_0*m_2 + l_2^2*m_1*m_2 - l_2^2*m_2^2*cos(y(3))^2))/(I_2*L_1^2*m_2^2 + I_2*l_1^2*m_1^2 + I_1*l_2^2*m_2^2 + I_1*I_2*m_0 + I_1*I_2*m_1 + I_1*I_2*m_2 + L_1^2*l_2^2*m_2^3 + L_1^2*l_2^2*m_0*m_2^2 + L_1^2*l_2^2*m_1*m_2^2 - L_1^2*l_2^2*m_2^3*cos(y(2) - y(3))^2 + I_2*L_1^2*m_0*m_2 + I_2*L_1^2*m_1*m_2 + l_1^2*l_2^2*m_1*m_2^2 + l_1^2*l_2^2*m_1^2*m_2 + I_2*l_1^2*m_0*m_1 + I_1*l_2^2*m_0*m_2 + I_1*l_2^2*m_1*m_2 + I_2*l_1^2*m_1*m_2 - I_2*L_1^2*m_2^2*cos(y(2))^2 - I_2*l_1^2*m_1^2*cos(y(2))^2 - I_1*l_2^2*m_2^2*cos(y(3))^2 - L_1^2*l_2^2*m_2^3*cos(y(2))^2 - L_1^2*l_2^2*m_2^3*cos(y(3))^2 + l_1^2*l_2^2*m_0*m_1*m_2 - l_1^2*l_2^2*m_1^2*m_2*cos(y(2))^2 - l_1^2*l_2^2*m_1*m_2^2*cos(y(3))^2 - L_1^2*l_2^2*m_0*m_2^2*cos(y(2) - y(3))^2 - L_1^2*l_2^2*m_1*m_2^2*cos(y(2) - y(3))^2 - 2*L_1*l_1*l_2^2*m_1*m_2^2*cos(y(2))^2 + 2*L_1^2*l_2^2*m_2^3*cos(y(2) - y(3))*cos(y(2))*cos(y(3)) - 2*I_2*L_1*l_1*m_1*m_2*cos(y(2))^2 + 2*L_1*l_1*l_2^2*m_1*m_2^2*cos(y(2) - y(3))*cos(y(2))*cos(y(3))) - (l_2*m_2*y(6)*sin(y(3))*(L_1*l_2^2*m_2^2*cos(y(2)) + I_2*L_1*m_2*cos(y(2)) + I_2*l_1*m_1*cos(y(2)) - L_1*l_2^2*m_2^2*cos(y(2) - y(3))*cos(y(3)) + l_1*l_2^2*m_1*m_2*cos(y(2))))/(I_2*L_1^2*m_2^2 + I_2*l_1^2*m_1^2 + I_1*l_2^2*m_2^2 + I_1*I_2*m_0 + I_1*I_2*m_1 + I_1*I_2*m_2 + L_1^2*l_2^2*m_2^3 + L_1^2*l_2^2*m_0*m_2^2 + L_1^2*l_2^2*m_1*m_2^2 - L_1^2*l_2^2*m_2^3*cos(y(2) - y(3))^2 + I_2*L_1^2*m_0*m_2 + I_2*L_1^2*m_1*m_2 + l_1^2*l_2^2*m_1*m_2^2 + l_1^2*l_2^2*m_1^2*m_2 + I_2*l_1^2*m_0*m_1 + I_1*l_2^2*m_0*m_2 + I_1*l_2^2*m_1*m_2 + I_2*l_1^2*m_1*m_2 - I_2*L_1^2*m_2^2*cos(y(2))^2 - I_2*l_1^2*m_1^2*cos(y(2))^2 - I_1*l_2^2*m_2^2*cos(y(3))^2 - L_1^2*l_2^2*m_2^3*cos(y(2))^2 - L_1^2*l_2^2*m_2^3*cos(y(3))^2 + l_1^2*l_2^2*m_0*m_1*m_2 - l_1^2*l_2^2*m_1^2*m_2*cos(y(2))^2 - l_1^2*l_2^2*m_1*m_2^2*cos(y(3))^2 - L_1^2*l_2^2*m_0*m_2^2*cos(y(2) - y(3))^2 - L_1^2*l_2^2*m_1*m_2^2*cos(y(2) - y(3))^2 - 2*L_1*l_1*l_2^2*m_1*m_2^2*cos(y(2))^2 + 2*L_1^2*l_2^2*m_2^3*cos(y(2) - y(3))*cos(y(2))*cos(y(3)) - 2*I_2*L_1*l_1*m_1*m_2*cos(y(2))^2 + 2*L_1*l_1*l_2^2*m_1*m_2^2*cos(y(2) - y(3))*cos(y(2))*cos(y(3)))) - conj(y(5))*(((b_1 + b_2)*(I_2*m_0 + I_2*m_1 + I_2*m_2 + l_2^2*m_2^2 + l_2^2*m_0*m_2 + l_2^2*m_1*m_2 - l_2^2*m_2^2*cos(y(3))^2))/(I_2*L_1^2*m_2^2 + I_2*l_1^2*m_1^2 + I_1*l_2^2*m_2^2 + I_1*I_2*m_0 + I_1*I_2*m_1 + I_1*I_2*m_2 + L_1^2*l_2^2*m_2^3 + L_1^2*l_2^2*m_0*m_2^2 + L_1^2*l_2^2*m_1*m_2^2 - L_1^2*l_2^2*m_2^3*cos(y(2) - y(3))^2 + I_2*L_1^2*m_0*m_2 + I_2*L_1^2*m_1*m_2 + l_1^2*l_2^2*m_1*m_2^2 + l_1^2*l_2^2*m_1^2*m_2 + I_2*l_1^2*m_0*m_1 + I_1*l_2^2*m_0*m_2 + I_1*l_2^2*m_1*m_2 + I_2*l_1^2*m_1*m_2 - I_2*L_1^2*m_2^2*cos(y(2))^2 - I_2*l_1^2*m_1^2*cos(y(2))^2 - I_1*l_2^2*m_2^2*cos(y(3))^2 - L_1^2*l_2^2*m_2^3*cos(y(2))^2 - L_1^2*l_2^2*m_2^3*cos(y(3))^2 + l_1^2*l_2^2*m_0*m_1*m_2 - l_1^2*l_2^2*m_1^2*m_2*cos(y(2))^2 - l_1^2*l_2^2*m_1*m_2^2*cos(y(3))^2 - L_1^2*l_2^2*m_0*m_2^2*cos(y(2) - y(3))^2 - L_1^2*l_2^2*m_1*m_2^2*cos(y(2) - y(3))^2 - 2*L_1*l_1*l_2^2*m_1*m_2^2*cos(y(2))^2 + 2*L_1^2*l_2^2*m_2^3*cos(y(2) - y(3))*cos(y(2))*cos(y(3)) - 2*I_2*L_1*l_1*m_1*m_2*cos(y(2))^2 + 2*L_1*l_1*l_2^2*m_1*m_2^2*cos(y(2) - y(3))*cos(y(2))*cos(y(3))) + ((b_2 + L_1*l_2*m_2*sin(y(2) - y(3))*y(5))*(L_1*l_2*m_2^2*cos(y(2) - y(3)) + L_1*l_2*m_0*m_2*cos(y(2) - y(3)) + L_1*l_2*m_1*m_2*cos(y(2) - y(3)) - L_1*l_2*m_2^2*cos(y(2))*cos(y(3)) - l_1*l_2*m_1*m_2*cos(y(2))*cos(y(3))))/(I_2*L_1^2*m_2^2 + I_2*l_1^2*m_1^2 + I_1*l_2^2*m_2^2 + I_1*I_2*m_0 + I_1*I_2*m_1 + I_1*I_2*m_2 + L_1^2*l_2^2*m_2^3 + L_1^2*l_2^2*m_0*m_2^2 + L_1^2*l_2^2*m_1*m_2^2 - L_1^2*l_2^2*m_2^3*cos(y(2) - y(3))^2 + I_2*L_1^2*m_0*m_2 + I_2*L_1^2*m_1*m_2 + l_1^2*l_2^2*m_1*m_2^2 + l_1^2*l_2^2*m_1^2*m_2 + I_2*l_1^2*m_0*m_1 + I_1*l_2^2*m_0*m_2 + I_1*l_2^2*m_1*m_2 + I_2*l_1^2*m_1*m_2 - I_2*L_1^2*m_2^2*cos(y(2))^2 - I_2*l_1^2*m_1^2*cos(y(2))^2 - I_1*l_2^2*m_2^2*cos(y(3))^2 - L_1^2*l_2^2*m_2^3*cos(y(2))^2 - L_1^2*l_2^2*m_2^3*cos(y(3))^2 + l_1^2*l_2^2*m_0*m_1*m_2 - l_1^2*l_2^2*m_1^2*m_2*cos(y(2))^2 - l_1^2*l_2^2*m_1*m_2^2*cos(y(3))^2 - L_1^2*l_2^2*m_0*m_2^2*cos(y(2) - y(3))^2 - L_1^2*l_2^2*m_1*m_2^2*cos(y(2) - y(3))^2 - 2*L_1*l_1*l_2^2*m_1*m_2^2*cos(y(2))^2 + 2*L_1^2*l_2^2*m_2^3*cos(y(2) - y(3))*cos(y(2))*cos(y(3)) - 2*I_2*L_1*l_1*m_1*m_2*cos(y(2))^2 + 2*L_1*l_1*l_2^2*m_1*m_2^2*cos(y(2) - y(3))*cos(y(2))*cos(y(3))) + (y(5)*sin(y(2))*(L_1*m_2 + l_1*m_1)*(L_1*l_2^2*m_2^2*cos(y(2)) + I_2*L_1*m_2*cos(y(2)) + I_2*l_1*m_1*cos(y(2)) - L_1*l_2^2*m_2^2*cos(y(2) - y(3))*cos(y(3)) + l_1*l_2^2*m_1*m_2*cos(y(2))))/(I_2*L_1^2*m_2^2 + I_2*l_1^2*m_1^2 + I_1*l_2^2*m_2^2 + I_1*I_2*m_0 + I_1*I_2*m_1 + I_1*I_2*m_2 + L_1^2*l_2^2*m_2^3 + L_1^2*l_2^2*m_0*m_2^2 + L_1^2*l_2^2*m_1*m_2^2 - L_1^2*l_2^2*m_2^3*cos(y(2) - y(3))^2 + I_2*L_1^2*m_0*m_2 + I_2*L_1^2*m_1*m_2 + l_1^2*l_2^2*m_1*m_2^2 + l_1^2*l_2^2*m_1^2*m_2 + I_2*l_1^2*m_0*m_1 + I_1*l_2^2*m_0*m_2 + I_1*l_2^2*m_1*m_2 + I_2*l_1^2*m_1*m_2 - I_2*L_1^2*m_2^2*cos(y(2))^2 - I_2*l_1^2*m_1^2*cos(y(2))^2 - I_1*l_2^2*m_2^2*cos(y(3))^2 - L_1^2*l_2^2*m_2^3*cos(y(2))^2 - L_1^2*l_2^2*m_2^3*cos(y(3))^2 + l_1^2*l_2^2*m_0*m_1*m_2 - l_1^2*l_2^2*m_1^2*m_2*cos(y(2))^2 - l_1^2*l_2^2*m_1*m_2^2*cos(y(3))^2 - L_1^2*l_2^2*m_0*m_2^2*cos(y(2) - y(3))^2 - L_1^2*l_2^2*m_1*m_2^2*cos(y(2) - y(3))^2 - 2*L_1*l_1*l_2^2*m_1*m_2^2*cos(y(2))^2 + 2*L_1^2*l_2^2*m_2^3*cos(y(2) - y(3))*cos(y(2))*cos(y(3)) - 2*I_2*L_1*l_1*m_1*m_2*cos(y(2))^2 + 2*L_1*l_1*l_2^2*m_1*m_2^2*cos(y(2) - y(3))*cos(y(2))*cos(y(3)))) - (u*(L_1*l_2^2*m_2^2*cos(y(2)) + I_2*L_1*m_2*cos(y(2)) + I_2*l_1*m_1*cos(y(2)) - L_1*l_2^2*m_2^2*cos(y(2) - y(3))*cos(y(3)) + l_1*l_2^2*m_1*m_2*cos(y(2))))/(I_2*L_1^2*m_2^2 + I_2*l_1^2*m_1^2 + I_1*l_2^2*m_2^2 + I_1*I_2*m_0 + I_1*I_2*m_1 + I_1*I_2*m_2 + L_1^2*l_2^2*m_2^3 + L_1^2*l_2^2*m_0*m_2^2 + L_1^2*l_2^2*m_1*m_2^2 - L_1^2*l_2^2*m_2^3*cos(y(2) - y(3))^2 + I_2*L_1^2*m_0*m_2 + I_2*L_1^2*m_1*m_2 + l_1^2*l_2^2*m_1*m_2^2 + l_1^2*l_2^2*m_1^2*m_2 + I_2*l_1^2*m_0*m_1 + I_1*l_2^2*m_0*m_2 + I_1*l_2^2*m_1*m_2 + I_2*l_1^2*m_1*m_2 - I_2*L_1^2*m_2^2*cos(y(2))^2 - I_2*l_1^2*m_1^2*cos(y(2))^2 - I_1*l_2^2*m_2^2*cos(y(3))^2 - L_1^2*l_2^2*m_2^3*cos(y(2))^2 - L_1^2*l_2^2*m_2^3*cos(y(3))^2 + l_1^2*l_2^2*m_0*m_1*m_2 - l_1^2*l_2^2*m_1^2*m_2*cos(y(2))^2 - l_1^2*l_2^2*m_1*m_2^2*cos(y(3))^2 - L_1^2*l_2^2*m_0*m_2^2*cos(y(2) - y(3))^2 - L_1^2*l_2^2*m_1*m_2^2*cos(y(2) - y(3))^2 - 2*L_1*l_1*l_2^2*m_1*m_2^2*cos(y(2))^2 + 2*L_1^2*l_2^2*m_2^3*cos(y(2) - y(3))*cos(y(2))*cos(y(3)) - 2*I_2*L_1*l_1*m_1*m_2*cos(y(2))^2 + 2*L_1*l_1*l_2^2*m_1*m_2^2*cos(y(2) - y(3))*cos(y(2))*cos(y(3))) + (b_0*conj(y(4))*(L_1*l_2^2*m_2^2*cos(y(2)) + I_2*L_1*m_2*cos(y(2)) + I_2*l_1*m_1*cos(y(2)) - L_1*l_2^2*m_2^2*cos(y(2) - y(3))*cos(y(3)) + l_1*l_2^2*m_1*m_2*cos(y(2))))/(I_2*L_1^2*m_2^2 + I_2*l_1^2*m_1^2 + I_1*l_2^2*m_2^2 + I_1*I_2*m_0 + I_1*I_2*m_1 + I_1*I_2*m_2 + L_1^2*l_2^2*m_2^3 + L_1^2*l_2^2*m_0*m_2^2 + L_1^2*l_2^2*m_1*m_2^2 - L_1^2*l_2^2*m_2^3*cos(y(2) - y(3))^2 + I_2*L_1^2*m_0*m_2 + I_2*L_1^2*m_1*m_2 + l_1^2*l_2^2*m_1*m_2^2 + l_1^2*l_2^2*m_1^2*m_2 + I_2*l_1^2*m_0*m_1 + I_1*l_2^2*m_0*m_2 + I_1*l_2^2*m_1*m_2 + I_2*l_1^2*m_1*m_2 - I_2*L_1^2*m_2^2*cos(y(2))^2 - I_2*l_1^2*m_1^2*cos(y(2))^2 - I_1*l_2^2*m_2^2*cos(y(3))^2 - L_1^2*l_2^2*m_2^3*cos(y(2))^2 - L_1^2*l_2^2*m_2^3*cos(y(3))^2 + l_1^2*l_2^2*m_0*m_1*m_2 - l_1^2*l_2^2*m_1^2*m_2*cos(y(2))^2 - l_1^2*l_2^2*m_1*m_2^2*cos(y(3))^2 - L_1^2*l_2^2*m_0*m_2^2*cos(y(2) - y(3))^2 - L_1^2*l_2^2*m_1*m_2^2*cos(y(2) - y(3))^2 - 2*L_1*l_1*l_2^2*m_1*m_2^2*cos(y(2))^2 + 2*L_1^2*l_2^2*m_2^3*cos(y(2) - y(3))*cos(y(2))*cos(y(3)) - 2*I_2*L_1*l_1*m_1*m_2*cos(y(2))^2 + 2*L_1*l_1*l_2^2*m_1*m_2^2*cos(y(2) - y(3))*cos(y(2))*cos(y(3))) + (g*sin(y(2))*(L_1*m_2 + l_1*m_1)*(I_2*m_0 + I_2*m_1 + I_2*m_2 + l_2^2*m_2^2 + l_2^2*m_0*m_2 + l_2^2*m_1*m_2 - l_2^2*m_2^2*cos(y(3))^2))/(I_2*L_1^2*m_2^2 + I_2*l_1^2*m_1^2 + I_1*l_2^2*m_2^2 + I_1*I_2*m_0 + I_1*I_2*m_1 + I_1*I_2*m_2 + L_1^2*l_2^2*m_2^3 + L_1^2*l_2^2*m_0*m_2^2 + L_1^2*l_2^2*m_1*m_2^2 - L_1^2*l_2^2*m_2^3*cos(y(2) - y(3))^2 + I_2*L_1^2*m_0*m_2 + I_2*L_1^2*m_1*m_2 + l_1^2*l_2^2*m_1*m_2^2 + l_1^2*l_2^2*m_1^2*m_2 + I_2*l_1^2*m_0*m_1 + I_1*l_2^2*m_0*m_2 + I_1*l_2^2*m_1*m_2 + I_2*l_1^2*m_1*m_2 - I_2*L_1^2*m_2^2*cos(y(2))^2 - I_2*l_1^2*m_1^2*cos(y(2))^2 - I_1*l_2^2*m_2^2*cos(y(3))^2 - L_1^2*l_2^2*m_2^3*cos(y(2))^2 - L_1^2*l_2^2*m_2^3*cos(y(3))^2 + l_1^2*l_2^2*m_0*m_1*m_2 - l_1^2*l_2^2*m_1^2*m_2*cos(y(2))^2 - l_1^2*l_2^2*m_1*m_2^2*cos(y(3))^2 - L_1^2*l_2^2*m_0*m_2^2*cos(y(2) - y(3))^2 - L_1^2*l_2^2*m_1*m_2^2*cos(y(2) - y(3))^2 - 2*L_1*l_1*l_2^2*m_1*m_2^2*cos(y(2))^2 + 2*L_1^2*l_2^2*m_2^3*cos(y(2) - y(3))*cos(y(2))*cos(y(3)) - 2*I_2*L_1*l_1*m_1*m_2*cos(y(2))^2 + 2*L_1*l_1*l_2^2*m_1*m_2^2*cos(y(2) - y(3))*cos(y(2))*cos(y(3))) - (g*l_2*m_2*sin(y(3))*(L_1*l_2*m_2^2*cos(y(2) - y(3)) + L_1*l_2*m_0*m_2*cos(y(2) - y(3)) + L_1*l_2*m_1*m_2*cos(y(2) - y(3)) - L_1*l_2*m_2^2*cos(y(2))*cos(y(3)) - l_1*l_2*m_1*m_2*cos(y(2))*cos(y(3))))/(I_2*L_1^2*m_2^2 + I_2*l_1^2*m_1^2 + I_1*l_2^2*m_2^2 + I_1*I_2*m_0 + I_1*I_2*m_1 + I_1*I_2*m_2 + L_1^2*l_2^2*m_2^3 + L_1^2*l_2^2*m_0*m_2^2 + L_1^2*l_2^2*m_1*m_2^2 - L_1^2*l_2^2*m_2^3*cos(y(2) - y(3))^2 + I_2*L_1^2*m_0*m_2 + I_2*L_1^2*m_1*m_2 + l_1^2*l_2^2*m_1*m_2^2 + l_1^2*l_2^2*m_1^2*m_2 + I_2*l_1^2*m_0*m_1 + I_1*l_2^2*m_0*m_2 + I_1*l_2^2*m_1*m_2 + I_2*l_1^2*m_1*m_2 - I_2*L_1^2*m_2^2*cos(y(2))^2 - I_2*l_1^2*m_1^2*cos(y(2))^2 - I_1*l_2^2*m_2^2*cos(y(3))^2 - L_1^2*l_2^2*m_2^3*cos(y(2))^2 - L_1^2*l_2^2*m_2^3*cos(y(3))^2 + l_1^2*l_2^2*m_0*m_1*m_2 - l_1^2*l_2^2*m_1^2*m_2*cos(y(2))^2 - l_1^2*l_2^2*m_1*m_2^2*cos(y(3))^2 - L_1^2*l_2^2*m_0*m_2^2*cos(y(2) - y(3))^2 - L_1^2*l_2^2*m_1*m_2^2*cos(y(2) - y(3))^2 - 2*L_1*l_1*l_2^2*m_1*m_2^2*cos(y(2))^2 + 2*L_1^2*l_2^2*m_2^3*cos(y(2) - y(3))*cos(y(2))*cos(y(3)) - 2*I_2*L_1*l_1*m_1*m_2*cos(y(2))^2 + 2*L_1*l_1*l_2^2*m_1*m_2^2*cos(y(2) - y(3))*cos(y(2))*cos(y(3))); 
dx(6) = conj(y(5))*(((b_1 + b_2)*(L_1*l_2*m_2^2*cos(y(2) - y(3)) + L_1*l_2*m_0*m_2*cos(y(2) - y(3)) + L_1*l_2*m_1*m_2*cos(y(2) - y(3)) - L_1*l_2*m_2^2*cos(y(2))*cos(y(3)) - l_1*l_2*m_1*m_2*cos(y(2))*cos(y(3))))/(I_2*L_1^2*m_2^2 + I_2*l_1^2*m_1^2 + I_1*l_2^2*m_2^2 + I_1*I_2*m_0 + I_1*I_2*m_1 + I_1*I_2*m_2 + L_1^2*l_2^2*m_2^3 + L_1^2*l_2^2*m_0*m_2^2 + L_1^2*l_2^2*m_1*m_2^2 - L_1^2*l_2^2*m_2^3*cos(y(2) - y(3))^2 + I_2*L_1^2*m_0*m_2 + I_2*L_1^2*m_1*m_2 + l_1^2*l_2^2*m_1*m_2^2 + l_1^2*l_2^2*m_1^2*m_2 + I_2*l_1^2*m_0*m_1 + I_1*l_2^2*m_0*m_2 + I_1*l_2^2*m_1*m_2 + I_2*l_1^2*m_1*m_2 - I_2*L_1^2*m_2^2*cos(y(2))^2 - I_2*l_1^2*m_1^2*cos(y(2))^2 - I_1*l_2^2*m_2^2*cos(y(3))^2 - L_1^2*l_2^2*m_2^3*cos(y(2))^2 - L_1^2*l_2^2*m_2^3*cos(y(3))^2 + l_1^2*l_2^2*m_0*m_1*m_2 - l_1^2*l_2^2*m_1^2*m_2*cos(y(2))^2 - l_1^2*l_2^2*m_1*m_2^2*cos(y(3))^2 - L_1^2*l_2^2*m_0*m_2^2*cos(y(2) - y(3))^2 - L_1^2*l_2^2*m_1*m_2^2*cos(y(2) - y(3))^2 - 2*L_1*l_1*l_2^2*m_1*m_2^2*cos(y(2))^2 + 2*L_1^2*l_2^2*m_2^3*cos(y(2) - y(3))*cos(y(2))*cos(y(3)) - 2*I_2*L_1*l_1*m_1*m_2*cos(y(2))^2 + 2*L_1*l_1*l_2^2*m_1*m_2^2*cos(y(2) - y(3))*cos(y(2))*cos(y(3))) + ((b_2 + L_1*l_2*m_2*sin(y(2) - y(3))*y(5))*(I_1*m_0 + I_1*m_1 + I_1*m_2 + L_1^2*m_2^2 + l_1^2*m_1^2 + l_1^2*m_0*m_1 + l_1^2*m_1*m_2 - L_1^2*m_2^2*cos(y(2))^2 - l_1^2*m_1^2*cos(y(2))^2 + L_1^2*m_0*m_2 + L_1^2*m_1*m_2 - 2*L_1*l_1*m_1*m_2*cos(y(2))^2))/(I_2*L_1^2*m_2^2 + I_2*l_1^2*m_1^2 + I_1*l_2^2*m_2^2 + I_1*I_2*m_0 + I_1*I_2*m_1 + I_1*I_2*m_2 + L_1^2*l_2^2*m_2^3 + L_1^2*l_2^2*m_0*m_2^2 + L_1^2*l_2^2*m_1*m_2^2 - L_1^2*l_2^2*m_2^3*cos(y(2) - y(3))^2 + I_2*L_1^2*m_0*m_2 + I_2*L_1^2*m_1*m_2 + l_1^2*l_2^2*m_1*m_2^2 + l_1^2*l_2^2*m_1^2*m_2 + I_2*l_1^2*m_0*m_1 + I_1*l_2^2*m_0*m_2 + I_1*l_2^2*m_1*m_2 + I_2*l_1^2*m_1*m_2 - I_2*L_1^2*m_2^2*cos(y(2))^2 - I_2*l_1^2*m_1^2*cos(y(2))^2 - I_1*l_2^2*m_2^2*cos(y(3))^2 - L_1^2*l_2^2*m_2^3*cos(y(2))^2 - L_1^2*l_2^2*m_2^3*cos(y(3))^2 + l_1^2*l_2^2*m_0*m_1*m_2 - l_1^2*l_2^2*m_1^2*m_2*cos(y(2))^2 - l_1^2*l_2^2*m_1*m_2^2*cos(y(3))^2 - L_1^2*l_2^2*m_0*m_2^2*cos(y(2) - y(3))^2 - L_1^2*l_2^2*m_1*m_2^2*cos(y(2) - y(3))^2 - 2*L_1*l_1*l_2^2*m_1*m_2^2*cos(y(2))^2 + 2*L_1^2*l_2^2*m_2^3*cos(y(2) - y(3))*cos(y(2))*cos(y(3)) - 2*I_2*L_1*l_1*m_1*m_2*cos(y(2))^2 + 2*L_1*l_1*l_2^2*m_1*m_2^2*cos(y(2) - y(3))*cos(y(2))*cos(y(3))) - (y(5)*sin(y(2))*(L_1*m_2 + l_1*m_1)*(L_1^2*l_2*m_2^2*cos(y(3)) + I_1*l_2*m_2*cos(y(3)) - L_1^2*l_2*m_2^2*cos(y(2) - y(3))*cos(y(2)) + l_1^2*l_2*m_1*m_2*cos(y(3)) - L_1*l_1*l_2*m_1*m_2*cos(y(2) - y(3))*cos(y(2))))/(I_2*L_1^2*m_2^2 + I_2*l_1^2*m_1^2 + I_1*l_2^2*m_2^2 + I_1*I_2*m_0 + I_1*I_2*m_1 + I_1*I_2*m_2 + L_1^2*l_2^2*m_2^3 + L_1^2*l_2^2*m_0*m_2^2 + L_1^2*l_2^2*m_1*m_2^2 - L_1^2*l_2^2*m_2^3*cos(y(2) - y(3))^2 + I_2*L_1^2*m_0*m_2 + I_2*L_1^2*m_1*m_2 + l_1^2*l_2^2*m_1*m_2^2 + l_1^2*l_2^2*m_1^2*m_2 + I_2*l_1^2*m_0*m_1 + I_1*l_2^2*m_0*m_2 + I_1*l_2^2*m_1*m_2 + I_2*l_1^2*m_1*m_2 - I_2*L_1^2*m_2^2*cos(y(2))^2 - I_2*l_1^2*m_1^2*cos(y(2))^2 - I_1*l_2^2*m_2^2*cos(y(3))^2 - L_1^2*l_2^2*m_2^3*cos(y(2))^2 - L_1^2*l_2^2*m_2^3*cos(y(3))^2 + l_1^2*l_2^2*m_0*m_1*m_2 - l_1^2*l_2^2*m_1^2*m_2*cos(y(2))^2 - l_1^2*l_2^2*m_1*m_2^2*cos(y(3))^2 - L_1^2*l_2^2*m_0*m_2^2*cos(y(2) - y(3))^2 - L_1^2*l_2^2*m_1*m_2^2*cos(y(2) - y(3))^2 - 2*L_1*l_1*l_2^2*m_1*m_2^2*cos(y(2))^2 + 2*L_1^2*l_2^2*m_2^3*cos(y(2) - y(3))*cos(y(2))*cos(y(3)) - 2*I_2*L_1*l_1*m_1*m_2*cos(y(2))^2 + 2*L_1*l_1*l_2^2*m_1*m_2^2*cos(y(2) - y(3))*cos(y(2))*cos(y(3)))) - conj(y(6))*((b_2*(I_1*m_0 + I_1*m_1 + I_1*m_2 + L_1^2*m_2^2 + l_1^2*m_1^2 + l_1^2*m_0*m_1 + l_1^2*m_1*m_2 - L_1^2*m_2^2*cos(y(2))^2 - l_1^2*m_1^2*cos(y(2))^2 + L_1^2*m_0*m_2 + L_1^2*m_1*m_2 - 2*L_1*l_1*m_1*m_2*cos(y(2))^2))/(I_2*L_1^2*m_2^2 + I_2*l_1^2*m_1^2 + I_1*l_2^2*m_2^2 + I_1*I_2*m_0 + I_1*I_2*m_1 + I_1*I_2*m_2 + L_1^2*l_2^2*m_2^3 + L_1^2*l_2^2*m_0*m_2^2 + L_1^2*l_2^2*m_1*m_2^2 - L_1^2*l_2^2*m_2^3*cos(y(2) - y(3))^2 + I_2*L_1^2*m_0*m_2 + I_2*L_1^2*m_1*m_2 + l_1^2*l_2^2*m_1*m_2^2 + l_1^2*l_2^2*m_1^2*m_2 + I_2*l_1^2*m_0*m_1 + I_1*l_2^2*m_0*m_2 + I_1*l_2^2*m_1*m_2 + I_2*l_1^2*m_1*m_2 - I_2*L_1^2*m_2^2*cos(y(2))^2 - I_2*l_1^2*m_1^2*cos(y(2))^2 - I_1*l_2^2*m_2^2*cos(y(3))^2 - L_1^2*l_2^2*m_2^3*cos(y(2))^2 - L_1^2*l_2^2*m_2^3*cos(y(3))^2 + l_1^2*l_2^2*m_0*m_1*m_2 - l_1^2*l_2^2*m_1^2*m_2*cos(y(2))^2 - l_1^2*l_2^2*m_1*m_2^2*cos(y(3))^2 - L_1^2*l_2^2*m_0*m_2^2*cos(y(2) - y(3))^2 - L_1^2*l_2^2*m_1*m_2^2*cos(y(2) - y(3))^2 - 2*L_1*l_1*l_2^2*m_1*m_2^2*cos(y(2))^2 + 2*L_1^2*l_2^2*m_2^3*cos(y(2) - y(3))*cos(y(2))*cos(y(3)) - 2*I_2*L_1*l_1*m_1*m_2*cos(y(2))^2 + 2*L_1*l_1*l_2^2*m_1*m_2^2*cos(y(2) - y(3))*cos(y(2))*cos(y(3))) + ((b_2 - L_1*l_2*m_2*sin(y(2) - y(3))*y(6))*(L_1*l_2*m_2^2*cos(y(2) - y(3)) + L_1*l_2*m_0*m_2*cos(y(2) - y(3)) + L_1*l_2*m_1*m_2*cos(y(2) - y(3)) - L_1*l_2*m_2^2*cos(y(2))*cos(y(3)) - l_1*l_2*m_1*m_2*cos(y(2))*cos(y(3))))/(I_2*L_1^2*m_2^2 + I_2*l_1^2*m_1^2 + I_1*l_2^2*m_2^2 + I_1*I_2*m_0 + I_1*I_2*m_1 + I_1*I_2*m_2 + L_1^2*l_2^2*m_2^3 + L_1^2*l_2^2*m_0*m_2^2 + L_1^2*l_2^2*m_1*m_2^2 - L_1^2*l_2^2*m_2^3*cos(y(2) - y(3))^2 + I_2*L_1^2*m_0*m_2 + I_2*L_1^2*m_1*m_2 + l_1^2*l_2^2*m_1*m_2^2 + l_1^2*l_2^2*m_1^2*m_2 + I_2*l_1^2*m_0*m_1 + I_1*l_2^2*m_0*m_2 + I_1*l_2^2*m_1*m_2 + I_2*l_1^2*m_1*m_2 - I_2*L_1^2*m_2^2*cos(y(2))^2 - I_2*l_1^2*m_1^2*cos(y(2))^2 - I_1*l_2^2*m_2^2*cos(y(3))^2 - L_1^2*l_2^2*m_2^3*cos(y(2))^2 - L_1^2*l_2^2*m_2^3*cos(y(3))^2 + l_1^2*l_2^2*m_0*m_1*m_2 - l_1^2*l_2^2*m_1^2*m_2*cos(y(2))^2 - l_1^2*l_2^2*m_1*m_2^2*cos(y(3))^2 - L_1^2*l_2^2*m_0*m_2^2*cos(y(2) - y(3))^2 - L_1^2*l_2^2*m_1*m_2^2*cos(y(2) - y(3))^2 - 2*L_1*l_1*l_2^2*m_1*m_2^2*cos(y(2))^2 + 2*L_1^2*l_2^2*m_2^3*cos(y(2) - y(3))*cos(y(2))*cos(y(3)) - 2*I_2*L_1*l_1*m_1*m_2*cos(y(2))^2 + 2*L_1*l_1*l_2^2*m_1*m_2^2*cos(y(2) - y(3))*cos(y(2))*cos(y(3))) + (l_2*m_2*y(6)*sin(y(3))*(L_1^2*l_2*m_2^2*cos(y(3)) + I_1*l_2*m_2*cos(y(3)) - L_1^2*l_2*m_2^2*cos(y(2) - y(3))*cos(y(2)) + l_1^2*l_2*m_1*m_2*cos(y(3)) - L_1*l_1*l_2*m_1*m_2*cos(y(2) - y(3))*cos(y(2))))/(I_2*L_1^2*m_2^2 + I_2*l_1^2*m_1^2 + I_1*l_2^2*m_2^2 + I_1*I_2*m_0 + I_1*I_2*m_1 + I_1*I_2*m_2 + L_1^2*l_2^2*m_2^3 + L_1^2*l_2^2*m_0*m_2^2 + L_1^2*l_2^2*m_1*m_2^2 - L_1^2*l_2^2*m_2^3*cos(y(2) - y(3))^2 + I_2*L_1^2*m_0*m_2 + I_2*L_1^2*m_1*m_2 + l_1^2*l_2^2*m_1*m_2^2 + l_1^2*l_2^2*m_1^2*m_2 + I_2*l_1^2*m_0*m_1 + I_1*l_2^2*m_0*m_2 + I_1*l_2^2*m_1*m_2 + I_2*l_1^2*m_1*m_2 - I_2*L_1^2*m_2^2*cos(y(2))^2 - I_2*l_1^2*m_1^2*cos(y(2))^2 - I_1*l_2^2*m_2^2*cos(y(3))^2 - L_1^2*l_2^2*m_2^3*cos(y(2))^2 - L_1^2*l_2^2*m_2^3*cos(y(3))^2 + l_1^2*l_2^2*m_0*m_1*m_2 - l_1^2*l_2^2*m_1^2*m_2*cos(y(2))^2 - l_1^2*l_2^2*m_1*m_2^2*cos(y(3))^2 - L_1^2*l_2^2*m_0*m_2^2*cos(y(2) - y(3))^2 - L_1^2*l_2^2*m_1*m_2^2*cos(y(2) - y(3))^2 - 2*L_1*l_1*l_2^2*m_1*m_2^2*cos(y(2))^2 + 2*L_1^2*l_2^2*m_2^3*cos(y(2) - y(3))*cos(y(2))*cos(y(3)) - 2*I_2*L_1*l_1*m_1*m_2*cos(y(2))^2 + 2*L_1*l_1*l_2^2*m_1*m_2^2*cos(y(2) - y(3))*cos(y(2))*cos(y(3)))) - (u*(L_1^2*l_2*m_2^2*cos(y(3)) + I_1*l_2*m_2*cos(y(3)) - L_1^2*l_2*m_2^2*cos(y(2) - y(3))*cos(y(2)) + l_1^2*l_2*m_1*m_2*cos(y(3)) - L_1*l_1*l_2*m_1*m_2*cos(y(2) - y(3))*cos(y(2))))/(I_2*L_1^2*m_2^2 + I_2*l_1^2*m_1^2 + I_1*l_2^2*m_2^2 + I_1*I_2*m_0 + I_1*I_2*m_1 + I_1*I_2*m_2 + L_1^2*l_2^2*m_2^3 + L_1^2*l_2^2*m_0*m_2^2 + L_1^2*l_2^2*m_1*m_2^2 - L_1^2*l_2^2*m_2^3*cos(y(2) - y(3))^2 + I_2*L_1^2*m_0*m_2 + I_2*L_1^2*m_1*m_2 + l_1^2*l_2^2*m_1*m_2^2 + l_1^2*l_2^2*m_1^2*m_2 + I_2*l_1^2*m_0*m_1 + I_1*l_2^2*m_0*m_2 + I_1*l_2^2*m_1*m_2 + I_2*l_1^2*m_1*m_2 - I_2*L_1^2*m_2^2*cos(y(2))^2 - I_2*l_1^2*m_1^2*cos(y(2))^2 - I_1*l_2^2*m_2^2*cos(y(3))^2 - L_1^2*l_2^2*m_2^3*cos(y(2))^2 - L_1^2*l_2^2*m_2^3*cos(y(3))^2 + l_1^2*l_2^2*m_0*m_1*m_2 - l_1^2*l_2^2*m_1^2*m_2*cos(y(2))^2 - l_1^2*l_2^2*m_1*m_2^2*cos(y(3))^2 - L_1^2*l_2^2*m_0*m_2^2*cos(y(2) - y(3))^2 - L_1^2*l_2^2*m_1*m_2^2*cos(y(2) - y(3))^2 - 2*L_1*l_1*l_2^2*m_1*m_2^2*cos(y(2))^2 + 2*L_1^2*l_2^2*m_2^3*cos(y(2) - y(3))*cos(y(2))*cos(y(3)) - 2*I_2*L_1*l_1*m_1*m_2*cos(y(2))^2 + 2*L_1*l_1*l_2^2*m_1*m_2^2*cos(y(2) - y(3))*cos(y(2))*cos(y(3))) + (b_0*conj(y(4))*(L_1^2*l_2*m_2^2*cos(y(3)) + I_1*l_2*m_2*cos(y(3)) - L_1^2*l_2*m_2^2*cos(y(2) - y(3))*cos(y(2)) + l_1^2*l_2*m_1*m_2*cos(y(3)) - L_1*l_1*l_2*m_1*m_2*cos(y(2) - y(3))*cos(y(2))))/(I_2*L_1^2*m_2^2 + I_2*l_1^2*m_1^2 + I_1*l_2^2*m_2^2 + I_1*I_2*m_0 + I_1*I_2*m_1 + I_1*I_2*m_2 + L_1^2*l_2^2*m_2^3 + L_1^2*l_2^2*m_0*m_2^2 + L_1^2*l_2^2*m_1*m_2^2 - L_1^2*l_2^2*m_2^3*cos(y(2) - y(3))^2 + I_2*L_1^2*m_0*m_2 + I_2*L_1^2*m_1*m_2 + l_1^2*l_2^2*m_1*m_2^2 + l_1^2*l_2^2*m_1^2*m_2 + I_2*l_1^2*m_0*m_1 + I_1*l_2^2*m_0*m_2 + I_1*l_2^2*m_1*m_2 + I_2*l_1^2*m_1*m_2 - I_2*L_1^2*m_2^2*cos(y(2))^2 - I_2*l_1^2*m_1^2*cos(y(2))^2 - I_1*l_2^2*m_2^2*cos(y(3))^2 - L_1^2*l_2^2*m_2^3*cos(y(2))^2 - L_1^2*l_2^2*m_2^3*cos(y(3))^2 + l_1^2*l_2^2*m_0*m_1*m_2 - l_1^2*l_2^2*m_1^2*m_2*cos(y(2))^2 - l_1^2*l_2^2*m_1*m_2^2*cos(y(3))^2 - L_1^2*l_2^2*m_0*m_2^2*cos(y(2) - y(3))^2 - L_1^2*l_2^2*m_1*m_2^2*cos(y(2) - y(3))^2 - 2*L_1*l_1*l_2^2*m_1*m_2^2*cos(y(2))^2 + 2*L_1^2*l_2^2*m_2^3*cos(y(2) - y(3))*cos(y(2))*cos(y(3)) - 2*I_2*L_1*l_1*m_1*m_2*cos(y(2))^2 + 2*L_1*l_1*l_2^2*m_1*m_2^2*cos(y(2) - y(3))*cos(y(2))*cos(y(3))) - (g*sin(y(2))*(L_1*m_2 + l_1*m_1)*(L_1*l_2*m_2^2*cos(y(2) - y(3)) + L_1*l_2*m_0*m_2*cos(y(2) - y(3)) + L_1*l_2*m_1*m_2*cos(y(2) - y(3)) - L_1*l_2*m_2^2*cos(y(2))*cos(y(3)) - l_1*l_2*m_1*m_2*cos(y(2))*cos(y(3))))/(I_2*L_1^2*m_2^2 + I_2*l_1^2*m_1^2 + I_1*l_2^2*m_2^2 + I_1*I_2*m_0 + I_1*I_2*m_1 + I_1*I_2*m_2 + L_1^2*l_2^2*m_2^3 + L_1^2*l_2^2*m_0*m_2^2 + L_1^2*l_2^2*m_1*m_2^2 - L_1^2*l_2^2*m_2^3*cos(y(2) - y(3))^2 + I_2*L_1^2*m_0*m_2 + I_2*L_1^2*m_1*m_2 + l_1^2*l_2^2*m_1*m_2^2 + l_1^2*l_2^2*m_1^2*m_2 + I_2*l_1^2*m_0*m_1 + I_1*l_2^2*m_0*m_2 + I_1*l_2^2*m_1*m_2 + I_2*l_1^2*m_1*m_2 - I_2*L_1^2*m_2^2*cos(y(2))^2 - I_2*l_1^2*m_1^2*cos(y(2))^2 - I_1*l_2^2*m_2^2*cos(y(3))^2 - L_1^2*l_2^2*m_2^3*cos(y(2))^2 - L_1^2*l_2^2*m_2^3*cos(y(3))^2 + l_1^2*l_2^2*m_0*m_1*m_2 - l_1^2*l_2^2*m_1^2*m_2*cos(y(2))^2 - l_1^2*l_2^2*m_1*m_2^2*cos(y(3))^2 - L_1^2*l_2^2*m_0*m_2^2*cos(y(2) - y(3))^2 - L_1^2*l_2^2*m_1*m_2^2*cos(y(2) - y(3))^2 - 2*L_1*l_1*l_2^2*m_1*m_2^2*cos(y(2))^2 + 2*L_1^2*l_2^2*m_2^3*cos(y(2) - y(3))*cos(y(2))*cos(y(3)) - 2*I_2*L_1*l_1*m_1*m_2*cos(y(2))^2 + 2*L_1*l_1*l_2^2*m_1*m_2^2*cos(y(2) - y(3))*cos(y(2))*cos(y(3))) + (g*l_2*m_2*sin(y(3))*(I_1*m_0 + I_1*m_1 + I_1*m_2 + L_1^2*m_2^2 + l_1^2*m_1^2 + l_1^2*m_0*m_1 + l_1^2*m_1*m_2 - L_1^2*m_2^2*cos(y(2))^2 - l_1^2*m_1^2*cos(y(2))^2 + L_1^2*m_0*m_2 + L_1^2*m_1*m_2 - 2*L_1*l_1*m_1*m_2*cos(y(2))^2))/(I_2*L_1^2*m_2^2 + I_2*l_1^2*m_1^2 + I_1*l_2^2*m_2^2 + I_1*I_2*m_0 + I_1*I_2*m_1 + I_1*I_2*m_2 + L_1^2*l_2^2*m_2^3 + L_1^2*l_2^2*m_0*m_2^2 + L_1^2*l_2^2*m_1*m_2^2 - L_1^2*l_2^2*m_2^3*cos(y(2) - y(3))^2 + I_2*L_1^2*m_0*m_2 + I_2*L_1^2*m_1*m_2 + l_1^2*l_2^2*m_1*m_2^2 + l_1^2*l_2^2*m_1^2*m_2 + I_2*l_1^2*m_0*m_1 + I_1*l_2^2*m_0*m_2 + I_1*l_2^2*m_1*m_2 + I_2*l_1^2*m_1*m_2 - I_2*L_1^2*m_2^2*cos(y(2))^2 - I_2*l_1^2*m_1^2*cos(y(2))^2 - I_1*l_2^2*m_2^2*cos(y(3))^2 - L_1^2*l_2^2*m_2^3*cos(y(2))^2 - L_1^2*l_2^2*m_2^3*cos(y(3))^2 + l_1^2*l_2^2*m_0*m_1*m_2 - l_1^2*l_2^2*m_1^2*m_2*cos(y(2))^2 - l_1^2*l_2^2*m_1*m_2^2*cos(y(3))^2 - L_1^2*l_2^2*m_0*m_2^2*cos(y(2) - y(3))^2 - L_1^2*l_2^2*m_1*m_2^2*cos(y(2) - y(3))^2 - 2*L_1*l_1*l_2^2*m_1*m_2^2*cos(y(2))^2 + 2*L_1^2*l_2^2*m_2^3*cos(y(2) - y(3))*cos(y(2))*cos(y(3)) - 2*I_2*L_1*l_1*m_1*m_2*cos(y(2))^2 + 2*L_1*l_1*l_2^2*m_1*m_2^2*cos(y(2) - y(3))*cos(y(2))*cos(y(3)));
